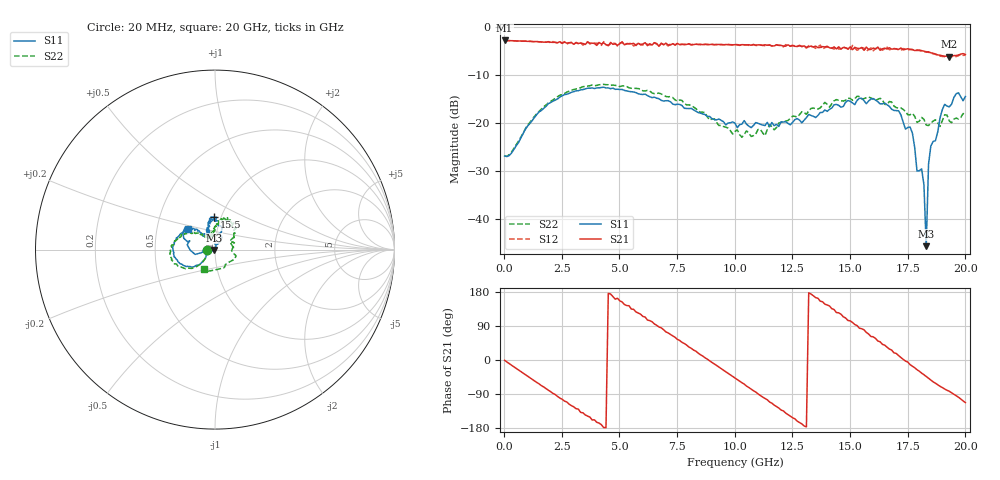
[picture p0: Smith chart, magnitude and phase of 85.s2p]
!Agilent Technologies,N5230A,US43500223,A.07.50.48
!Agilent N5230A: A.07.50.48
!Date: Monday, September 14, 2015 17:08:15
!Correction: S11(Full 2 Port(1,2))
!S21(Full 2 Port(1,2))
!S12(Full 2 Port(1,2))
!S22(Full 2 Port(1,2))
!S2P File: Measurements: S11, S21, S12, S22:
# Hz S  dB  R 50
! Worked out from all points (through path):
!   201 points, 20 MHz to 20 GHz, reference 50 ohm
!   highest |S21| = -2.80 dB at 20 MHz (marker M1); lowest = -6.2 dB at 19.3 GHz (marker M2)
!   group delay of S21, straight-line fit = 115 ps
!   lowest |S11| = -45.6 dB at 18.3 GHz (marker M3), VSWR 1.01, Z = 49.5 - j0.186 ohm
!   |S11| at or under -10 dB: start of sweep to end of sweep
!   |S22| runs from -26.9 to -11.9 dB; largest |S21 - S12| = 0.065
!   S11 on the Smith chart (normalised r, x): 20 MHz: 0.91, -0.00; 15.5 GHz: 0.93, +0.35; 20 GHz: 0.72, +0.17
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2e7  -26.83 -178.8  -2.80 -0.9  -2.79 -0.9  -26.79 -178.9
1.9181e9  -15.93 -142.4  -3.05 -79.8  -3.05 -80.2  -15.76 -140.3
3.4166e9  -13.00 -167.2  -3.43 -139.3  -3.77 -139.3  -12.40 -160.7
4.3157e9  -12.52 176.5  -3.28 -178.3  -3.04 -175.4  -11.92 -173.9
5.1149e9  -12.97 162.9  -3.07 153.1  -3.22 152.3  -12.25 175.7
6.7133e9  -14.90 139.7  -4.02 87.1  -3.94 87.6  -13.74 155.5
8.5115e9  -17.89 131.1  -3.58 13.9  -3.68 14.5  -17.73 133.9
1.001e10  -19.99 124.3  -3.66 -47.6  -3.64 -47.4  -21.72 120.6
1.15085e10  -20.73 114.0  -3.74 -110.7  -3.72 -109.5  -20.31 102.5
1.26074e10  -19.24 112.8  -4.02 -155.3  -3.85 -156.9  -18.56 92.4
1.34066e10  -18.56 106.5  -4.15 169.5  -4.13 167.8  -16.85 83.7
1.45055e10  -16.28 99.9  -4.11 124.5  -4.60 122.9  -15.23 79.2
1.55045e10  -14.82 91.4  -4.27 82.6  -4.27 82.4  -14.97 67.8
1.67033e10  -16.50 80.6  -4.31 29.0  -4.72 28.7  -15.49 46.9
1.77023e10  -22.07 60.3  -4.66 -16.4  -4.74 -16.3  -17.94 32.8
1.79021e10  -29.94 65.2  -4.79 -25.6  -4.87 -24.5  -19.84 30.7
1.82018e10  -32.75 73.8  -5.02 -38.8  -5.12 -38.7  -19.17 21.3
1.83017e10  -45.56 -159.1  -5.22 -43.4  -5.11 -43.9  -20.39 27.9
1.84016e10  -28.52 -153.0  -5.15 -48.3  -5.28 -48.6  -20.49 24.8
1.85015e10  -24.74 -166.9  -5.36 -52.5  -5.43 -52.8  -20.02 10.7
1.93007e10  -16.59 161.0  -6.19 -82.5  -6.29 -82.9  -19.53 -40.8
2e10  -14.44 143.1  -5.70 -112.3  -5.87 -112.3  -18.10 -118.1
